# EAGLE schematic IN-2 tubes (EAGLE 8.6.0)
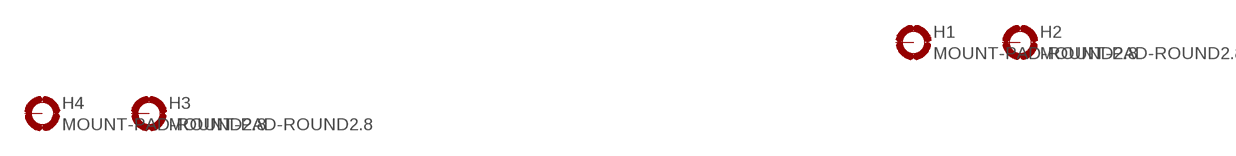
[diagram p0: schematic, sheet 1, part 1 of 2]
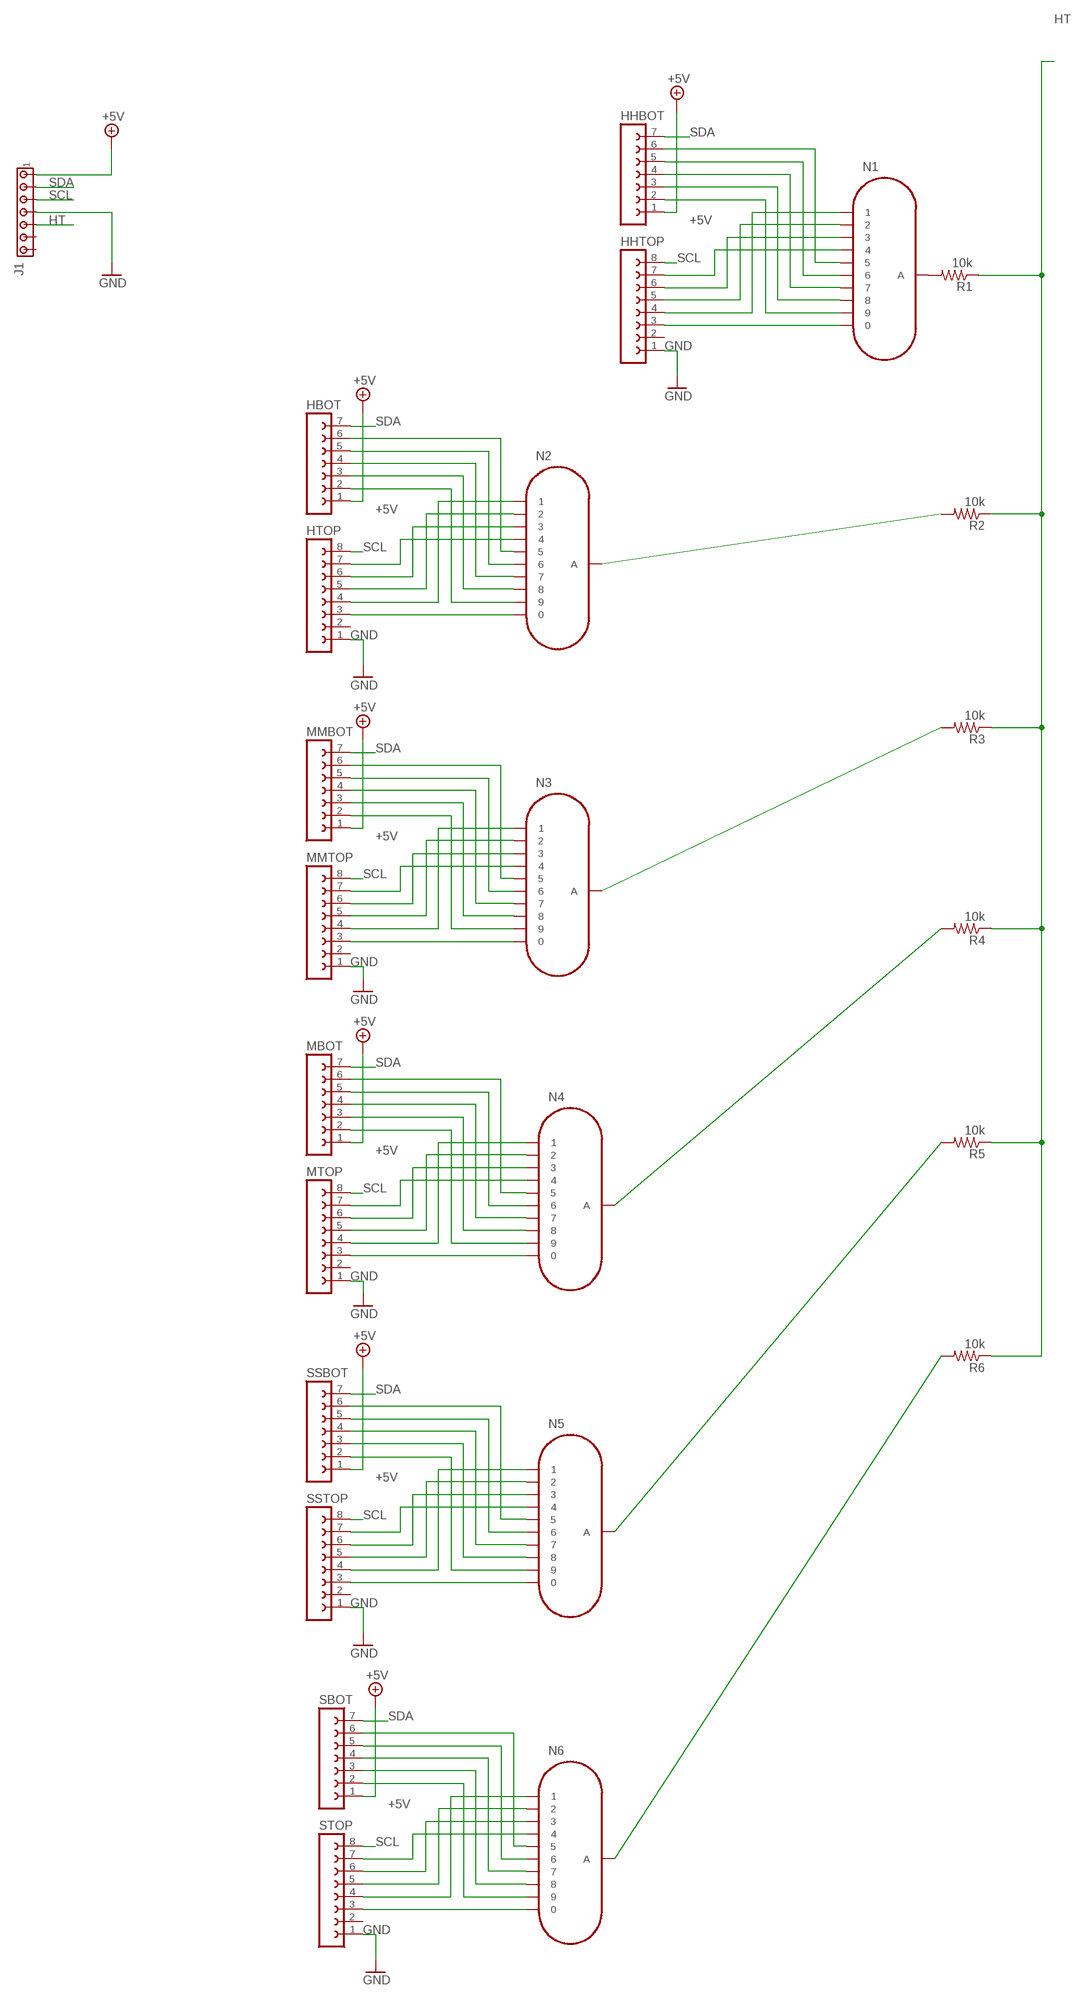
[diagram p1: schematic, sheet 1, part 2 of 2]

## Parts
H1  MOUNT-PAD-ROUND2.8  [2,8-PAD]
H2  MOUNT-PAD-ROUND2.8  [2,8-PAD]
H3  MOUNT-PAD-ROUND2.8  [2,8-PAD]
H4  MOUNT-PAD-ROUND2.8  [2,8-PAD]
HBOT  FE07-1  [FE07]
HHBOT  FE07-1  [FE07]
HHTOP  FE08-1  [FE08]
HTOP  FE08-1  [FE08]
J1  MTA07-100  [10X07MTA]
MBOT  FE07-1  [FE07]
MMBOT  FE07-1  [FE07]
MMTOP  FE08-1  [FE08]
MTOP  FE08-1  [FE08]
N1  IN-2  [IN-8]
N2  IN-2  [IN-8]
N3  IN-2  [IN-8]
N4  IN-2  [IN-8]
N5  IN-2  [IN-8]
N6  IN-2  [IN-8]
R1  10k  R-US_M0805  [M0805]
R2  10k  R-US_M0805  [M0805]
R3  10k  R-US_M0805  [M0805]
R4  10k  R-US_M0805  [M0805]
R5  10k  R-US_M0805  [M0805]
R6  10k  R-US_M0805  [M0805]
SBOT  FE07-1  [FE07]
SSBOT  FE07-1  [FE07]
SSTOP  FE08-1  [FE08]
STOP  FE08-1  [FE08]

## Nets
+5V: HBOT.1 HHBOT.1 J1.1 MBOT.1 MMBOT.1 SBOT.1 SSBOT.1
GND: HHTOP.1 HTOP.1 J1.4 MMTOP.1 MTOP.1 SSTOP.1 STOP.1
HT: J1.5 R1.1 R2.1 R3.1 R4.1 R5.1 R6.1
N$1: HHTOP.3 N1.0
N$2: HHTOP.4 N1.1
N$3: HHTOP.5 N1.2
N$4: HHTOP.6 N1.3
N$5: HHTOP.7 N1.4
N$6: HTOP.3 N2.0
N$7: HTOP.4 N2.1
N$8: HTOP.5 N2.2
N$9: N4.A R4.2
N$10: HTOP.6 N2.3
N$11: HTOP.7 N2.4
N$12: HBOT.6 N2.5
N$13: HBOT.5 N2.6
N$14: N2.A R2.2
N$15: HBOT.4 N2.7
N$16: HBOT.3 N2.8
N$17: N3.A R3.2
N$18: HBOT.2 N2.9
N$19: N6.A R6.2
N$20: N5.A R5.2
N$21: MMTOP.3 N3.0
N$22: N1.A R1.2
N$32: MMTOP.4 N3.1
N$33: MMTOP.5 N3.2
N$34: MMTOP.6 N3.3
N$35: MMTOP.7 N3.4
N$36: MMBOT.6 N3.5
N$37: MMBOT.5 N3.6
N$38: MMBOT.4 N3.7
N$39: MMBOT.3 N3.8
N$40: MMBOT.2 N3.9
N$41: MTOP.3 N4.0
N$42: MTOP.4 N4.1
N$43: MTOP.5 N4.2
N$44: MTOP.6 N4.3
N$45: MTOP.7 N4.4
N$46: MBOT.6 N4.5
N$47: MBOT.5 N4.6
N$48: MBOT.4 N4.7
N$49: MBOT.3 N4.8
N$51: MBOT.2 N4.9
N$52: N5.0 SSTOP.3
N$53: N5.1 SSTOP.4
N$54: N5.2 SSTOP.5
N$55: N5.3 SSTOP.6
N$56: N5.4 SSTOP.7
N$57: N5.5 SSBOT.6
N$58: N5.6 SSBOT.5
N$59: N5.7 SSBOT.4
N$60: N5.8 SSBOT.3
N$61: N5.9 SSBOT.2
N$62: N6.0 STOP.3
N$63: N6.1 STOP.4
N$64: N6.2 STOP.5
N$65: N6.3 STOP.6
N$66: N6.4 STOP.7
N$67: N6.5 SBOT.6
N$68: N6.6 SBOT.5
N$69: N6.7 SBOT.4
N$70: N6.8 SBOT.3
N$71: N6.9 SBOT.2
N$72: HHBOT.6 N1.5
N$73: HHBOT.5 N1.6
N$74: HHBOT.4 N1.7
N$75: HHBOT.3 N1.8
N$76: HHBOT.2 N1.9
SCL: HHTOP.8 HTOP.8 J1.3 MMTOP.8 MTOP.8 SSTOP.8 STOP.8
SDA: HBOT.7 HHBOT.7 J1.2 MBOT.7 MMBOT.7 SBOT.7 SSBOT.7
Unconnected: H1.B2,8(MOUNT) H2.B2,8(MOUNT) H3.B2,8(MOUNT) H4.B2,8(MOUNT) HHTOP.2 HTOP.2 J1.6 J1.7 MMTOP.2 MTOP.2 SSTOP.2 STOP.2

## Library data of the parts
H1-H4 = holes:MOUNT-PAD-ROUND: MOUNTING PAD, round
HBOT HHBOT MBOT MMBOT SBOT SSBOT = con-lsta:FE07-1: FEMALE HEADER; OC_FARNELL: unknown; OC_NEWARK: unknown
HHTOP HTOP MMTOP MTOP SSTOP STOP = con-lsta:FE08-1: FEMALE HEADER; OC_FARNELL: unknown; OC_NEWARK: unknown
J1 = con-amp:MTA07-100: AMP connector
N1-N6 = russian-nixies:IN-2: IN-2: tiny numeric topview nixie tube
R1-R6 = adafruit:R-US_: RESISTOR, American symbol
